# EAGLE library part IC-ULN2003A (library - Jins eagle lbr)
DRIVER ARRAY
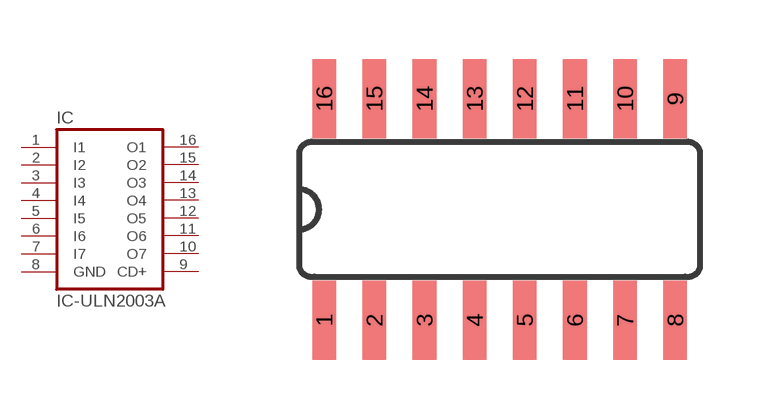
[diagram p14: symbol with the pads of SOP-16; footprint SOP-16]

Designator prefix IC

## IC-ULN2003AS  [SOP-16]
1  I1  in
2  I2  in
3  I3  in
4  I4  in
5  I5  in
6  I6  in
7  I7  in
8  GND  pwr
9  CD+  pas
10  O7  oc
11  O6  oc
12  O5  oc
13  O4  oc
14  O3  oc
15  O2  oc
16  O1  oc

## Footprint SOP-16 (pad centres in mm)
smd 0.6 x 2: 1 -3.945,-2.76; 2 -2.675,-2.76; 3 -1.405,-2.76; 4 -0.135,-2.76; 5 1.135,-2.76; 6 2.405,-2.76; 7 3.675,-2.76; 8 4.945,-2.76; 9 4.945,2.84; 10 3.675,2.84; 11 2.405,2.84; 12 1.135,2.84; 13 -0.135,2.84; 14 -1.405,2.84; 15 -2.675,2.84; 16 -3.945,2.84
